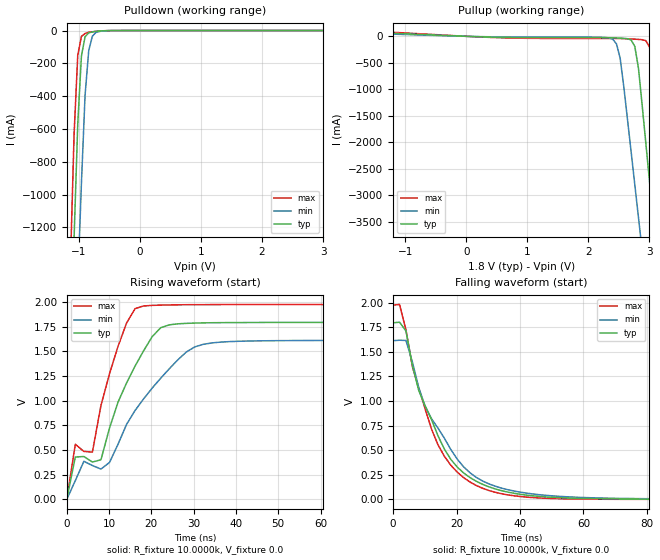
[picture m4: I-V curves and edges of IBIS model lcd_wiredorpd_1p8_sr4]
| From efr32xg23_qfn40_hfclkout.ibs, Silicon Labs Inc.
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|   Model lcd_wiredorpd_1p8_sr4
[Model]  lcd_wiredorpd_1p8_sr4
Model_type Output
Polarity   Non-Inverting
Enable   Active-Low
C_comp   1.6300pF   1.4000pF   2.7000pF
[Temperature Range]   25.0000   0.1250k   -40.0000
[Pullup Reference]   1.8000V   1.6200V   1.9800V
[Pulldown Reference]   0.0V   0.0V   0.0V
[POWER Clamp Reference]   1.8000V   1.6200V   1.9800V
[GND Clamp Reference]   0.0V   0.0V   0.0V
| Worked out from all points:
|   slope of the pulldown table from 0 to 0.27 V, typ, clamps not added: 40.6 kohm
|   slope of the pullup table from 0 to 0.27 V, typ, clamps not added: 26.3 ohm
|   rising waveform, R_fixture 10.0000k, V_fixture 0.0: 20-80 % time 15.6ns typ, 15ns min, 10.9ns max; typ from 0 V to 1.79 V
|   falling waveform, R_fixture 10.0000k, V_fixture 0.0: 20-80 % time 13.8ns typ, 15.6ns min, 12.3ns max; typ from 1.8 V to 0 V
[Pulldown]
|Voltage   I(typ)   I(min)   I(max)
-1.8V     -9.867A    -9.569A    -10.32A
-1.14V    -1.973A    -2.773A    -1.419A
-1.08V    -1.26A     -2.157A    -630.5mA
-1.02V    -568mA     -1.543A    -149.7mA
-960mV    -155.8mA   -930mA     -35.75mA
-900mV    -37.31mA   -392mA     -18.18mA
-840mV    -13.93mA   -121.5mA   -10.47mA
-780mV    -8.737mA   -34.04mA   -7.436mA
-720mV    -4.306mA   -11.22mA   -4.934mA
-660mV    -2.722mA   -5.276mA   -2.953mA
-360mV    -27.29uA   -76.51uA   -16.82uA
3.6V      88.26uA    75.14uA    103.4uA
[Pullup]
|Voltage   I(typ)   I(min)   I(max)
-1.8V     89.55mA    65.7mA     113.4mA
2.4V      -28.8mA    -55.09mA   -41.35mA
2.52V     -33.4mA    -414.8mA   -42.59mA
2.76V     -189.9mA   -2.797A    -53.83mA
2.82V     -601mA     -3.414A    -58.12mA
2.94V     -2.006A    -4.65A     -82.38mA
3V        -2.722A    -5.268A    -196.6mA
3.06V     -3.439A    -5.887A    -675.1mA
3.12V     -4.156A    -6.505A    -1.464A
3.24V     -5.593A    -7.743A    -3.076A
3.3V      -6.312A    -8.362A    -3.885A
3.6V      -9.909A    -11.46A    -7.939A
[Ramp]
| variable   typ   min   max
dV/dt_r  1.0773/15.5620n   0.9682/20.1386n   1.1859/10.9348n
dV/dt_f  0.2131/8.5758n   0.1690/11.9012n   0.2652/6.7990n
R_load = 10.0000k
[Rising Waveform]
R_fixture= 10.0000k
V_fixture= 0.0
V_fixture_min= 0.0
V_fixture_max= 0.0
|time   V(typ)   V(min)   V(max)
0s        2.578uV    44.87uV    2.149uV
2.02ns    429.2mV    190mV      558.7mV
4.04ns    434.3mV    385.5mV    485.8mV
6.061ns   378.2mV    342.8mV    479.1mV
8.081ns   401.5mV    307.1mV    952.3mV
14.14ns   1.181V     760.6mV    1.789V
18.18ns   1.508V     1.02V      1.962V
22.22ns   1.741V     1.229V     1.97V
36.36ns   1.792V     1.595V     1.976V
200ns     1.795V     1.614V     1.976V
[Falling Waveform]
R_fixture= 10.0000k
V_fixture= 0.0
V_fixture_min= 0.0
V_fixture_max= 0.0
|time   V(typ)   V(min)   V(max)
0s        1.796V     1.614V     1.977V
2.02ns    1.802V     1.619V     1.982V
4.04ns    1.713V     1.616V     1.722V
6.061ns   1.363V     1.397V     1.35V
8.081ns   1.105V     1.134V     1.131V
14.14ns   644.8mV    723.9mV    554mV
20.2ns    327.4mV    408.2mV    275.9mV
30.3ns    124.9mV    154.9mV    87.66mV
62.63ns   6.157mV    14.66mV    517.7uV
200ns     -87.29uV   581.7uV    -354.3uV
